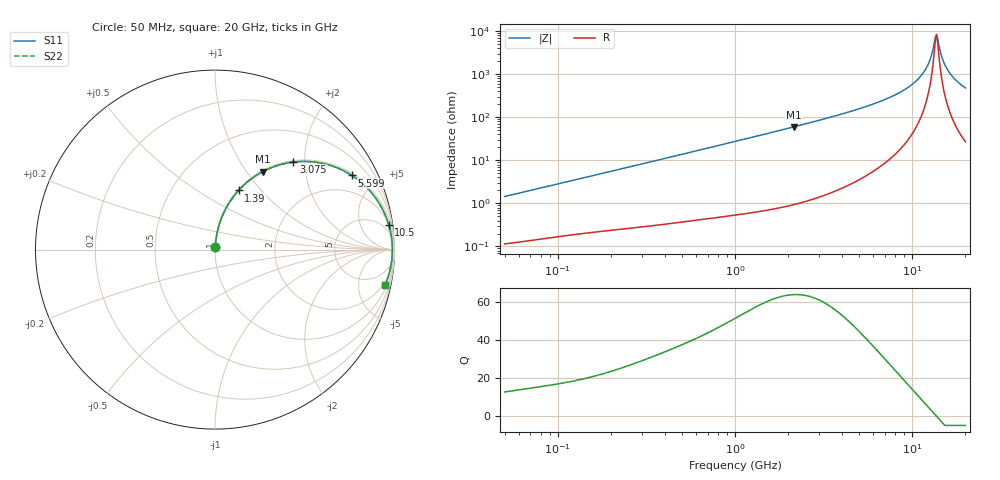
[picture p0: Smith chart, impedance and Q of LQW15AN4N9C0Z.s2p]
!Murata Part Number: LQW15AN4N9C0Z
!These Parameters are Measured in Series Mode Connection
!  o--[Z]--o
!Port1  Port2
!  o-------o
!Freq. Start=50[MHz] Stop=20[GHz], 401[Steps]
# Hz S RI R 50
!Freq.(Hz) S11(Real) S11(Imag) S21(Real) S21(Imag) S12(Real) S12(Imag) S22(Real) S22(Imag)
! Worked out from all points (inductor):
!   401 points, 50 MHz to 20 GHz, reference 50 ohm
!   read as one part in series: L = 4.57 nH near 51.52 MHz
!   highest Q = 63.7 at 2.147 GHz (marker M1), where L = 4.43 nH
!   self-resonance near 13.55 GHz
!   S11 on the Smith chart (normalised r, x): 50 MHz: 1.00, +0.03; 1.39 GHz: 1.01, +0.76; 3.075 GHz: 1.03, +1.76; 5.599 GHz: 1.09, +3.64; 10.5 GHz: 2, +14; 20 GHz: 1.54, -9.60
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5e7  0.00135 0.0144  0.9986 -0.0144  0.9986 -0.0144  0.00135 0.0144
1.364002e8  0.00344 0.0381  0.9966 -0.0381  0.9966 -0.0381  0.00344 0.0381
3.721004e8  0.0135 0.1009  0.9865 -0.1009  0.9865 -0.1009  0.0135 0.1009
1e9  0.074 0.2523  0.926 -0.2523  0.926 -0.2523  0.074 0.2523
1.390315e9  0.1315 0.3295  0.8685 -0.3295  0.8685 -0.3295  0.1315 0.3295
2.146657e9  0.2662 0.4342  0.7338 -0.4342  0.7338 -0.4342  0.2662 0.4342
2.728004e9  0.3745 0.476  0.6255 -0.476  0.6255 -0.476  0.3745 0.476
3.075291e9  0.4365 0.4877  0.5635 -0.4877  0.5635 -0.4877  0.4365 0.4877
5.598765e9  0.7627 0.4131  0.2373 -0.4131  0.2373 -0.4131  0.7627 0.4131
7.442007e9  0.8821 0.3047  0.1179 -0.3047  0.1179 -0.3047  0.8821 0.3047
9.041845e9  0.939 0.214  0.061 -0.214  0.061 -0.214  0.939 0.214
1.050288e10  0.968 0.139  0.032 -0.139  0.032 -0.139  0.968 0.139
1.149051e10  0.9793 0.0927  0.0207 -0.0927  0.0207 -0.0927  0.9793 0.0927
1.220001e10  0.9843 0.0615  0.0157 -0.0615  0.0157 -0.0615  0.9843 0.0615
1.276073e10  0.9867 0.038  0.0133 -0.038  0.0133 -0.038  0.9867 0.038
1.334722e10  0.988 0.0144  0.012 -0.0144  0.012 -0.0144  0.988 0.0144
1.375312e10  0.9882 -0.00133  0.0118 0.00133  0.0118 0.00133  0.9882 -0.00133
1.396067e10  0.9882 -0.00919  0.0118 0.00919  0.0118 0.00919  0.9882 -0.00919
1.504638e10  0.9859 -0.0485  0.0141 0.0485  0.0141 0.0485  0.9859 -0.0485
1.597544e10  0.9818 -0.0798  0.0182 0.0798  0.0182 0.0798  0.9818 -0.0798
1.774144e10  0.9698 -0.1341  0.0302 0.1341  0.0302 0.1341  0.9698 -0.1341
2e10  0.9485 -0.1946  0.0515 0.1946  0.0515 0.1946  0.9485 -0.1946
